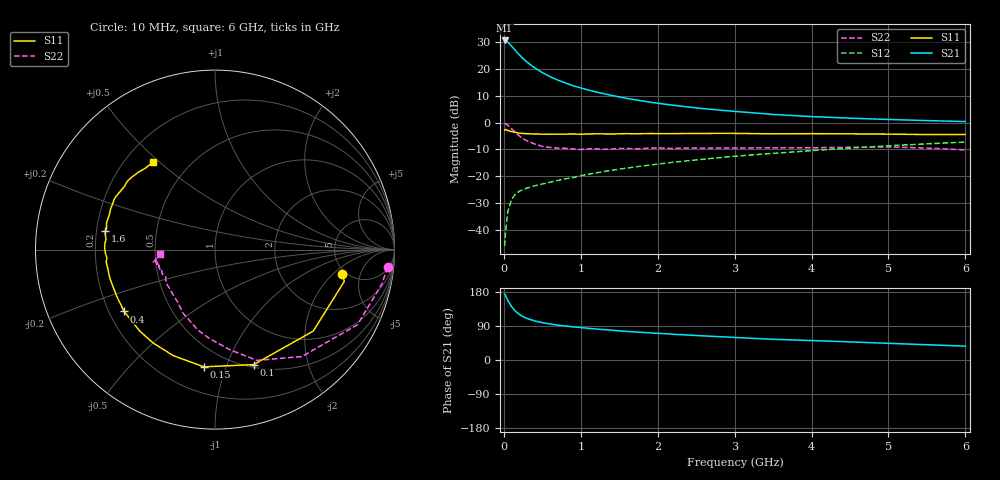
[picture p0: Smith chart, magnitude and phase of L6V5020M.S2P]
!  INFINEON TECHNOLOGIES Small Signal Semiconductors
! BFR380L3 , Si-NPN RF-Transistor in TSLP-3-1
!  Vce=0.5 V,  Ic=20 mA
! Common Emitter S-Parameters:  07. March 2005
#  GHz  S  MA  R  50
! f  S11  S21  S12  S22
! GHz  Mag  Ang  Mag  Ang  Mag  Ang  Mag  Ang
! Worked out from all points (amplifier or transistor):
!   36 points, 10 MHz to 6 GHz, reference 50 ohm
!   highest |S21| = 30.7 dB at 10 MHz (marker M1)
!   |S21| within 3 dB of that: start of sweep to 127.7 MHz
!   unconditionally stable (mu >= 1): 1.542 GHz to end of sweep
!   at 250 MHz: K = 0.40, MSG = 24.5 dB, |S12| = -25.0 dB
!   at 1.4 GHz: K = 0.99, MSG = 14.0 dB, |S12| = -17.9 dB
!   at 6 GHz: K = 1.00, MAG = 3.4 dB, |S12| = -7.3 dB
!   S11 on the Smith chart (normalised r, x): 10 MHz: 4.65, -2.62; 100 MHz: 0.53, -1.25; 150 MHz: 0.37, -0.84; 400 MHz: 0.26, -0.29; 1.6 GHz: 0.24, +0.08; 6 GHz: 0.31, +0.47
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0.01  0.7213 -10.8  34.15 173.7  0.0049 82.0  0.9668 -5.8
0.02  0.7419 -13.8  33.66 171.2  0.0083 80.9  0.949 -11.7
0.05  0.7111 -39.7  31.77 158.1  0.0213 72.5  0.8974 -27.8
0.1  0.676 -71.4  26.86 141.2  0.0365 60.0  0.7677 -50.9
0.15  0.6561 -95.4  22.21 128.8  0.0461 51.2  0.6604 -69.2
0.2  0.635 -111.4  18.49 120.5  0.0518 48.2  0.5658 -81.3
0.25  0.6242 -123.6  15.71 114.5  0.056 45.0  0.4968 -93.5
0.3  0.6179 -132.7  13.49 109.8  0.0598 44.1  0.4589 -101.9
0.4  0.6125 -145.8  10.53 103.1  0.0659 44.3  0.3961 -116.8
0.5  0.6062 -154.4  8.589 98.6  0.071 45.9  0.3585 -125.6
0.6  0.6049 -160.8  7.188 95.0  0.0767 47.5  0.3427 -133.0
0.7  0.6072 -165.0  6.229 92.2  0.0828 49.7  0.3327 -139.6
0.9  0.6104 -173.6  4.879 87.5  0.0937 52.5  0.321 -149.0
1.1  0.6114 -178.4  4.043 83.6  0.1082 55.0  0.3228 -153.1
1.3  0.6142 176.4  3.455 80.0  0.1215 56.5  0.3171 -159.3
1.6  0.6205 170.5  2.829 75.4  0.141 58.0  0.3277 -163.5
2.2  0.6199 161.7  2.107 68.0  0.1808 59.6  0.3273 -165.6
2.8  0.6278 153.6  1.709 61.6  0.2203 60.2  0.335 -169.2
3.5  0.6153 145.3  1.418 54.7  0.2654 58.3  0.3379 -169.0
4.5  0.6144 138.9  1.206 47.8  0.3335 56.5  0.3443 -169.0
5.5  0.5965 130.4  1.088 40.3  0.4001 52.2  0.3329 -170.9
6  0.5979 125.5  1.042 36.6  0.4328 49.9  0.3082 -175.8
